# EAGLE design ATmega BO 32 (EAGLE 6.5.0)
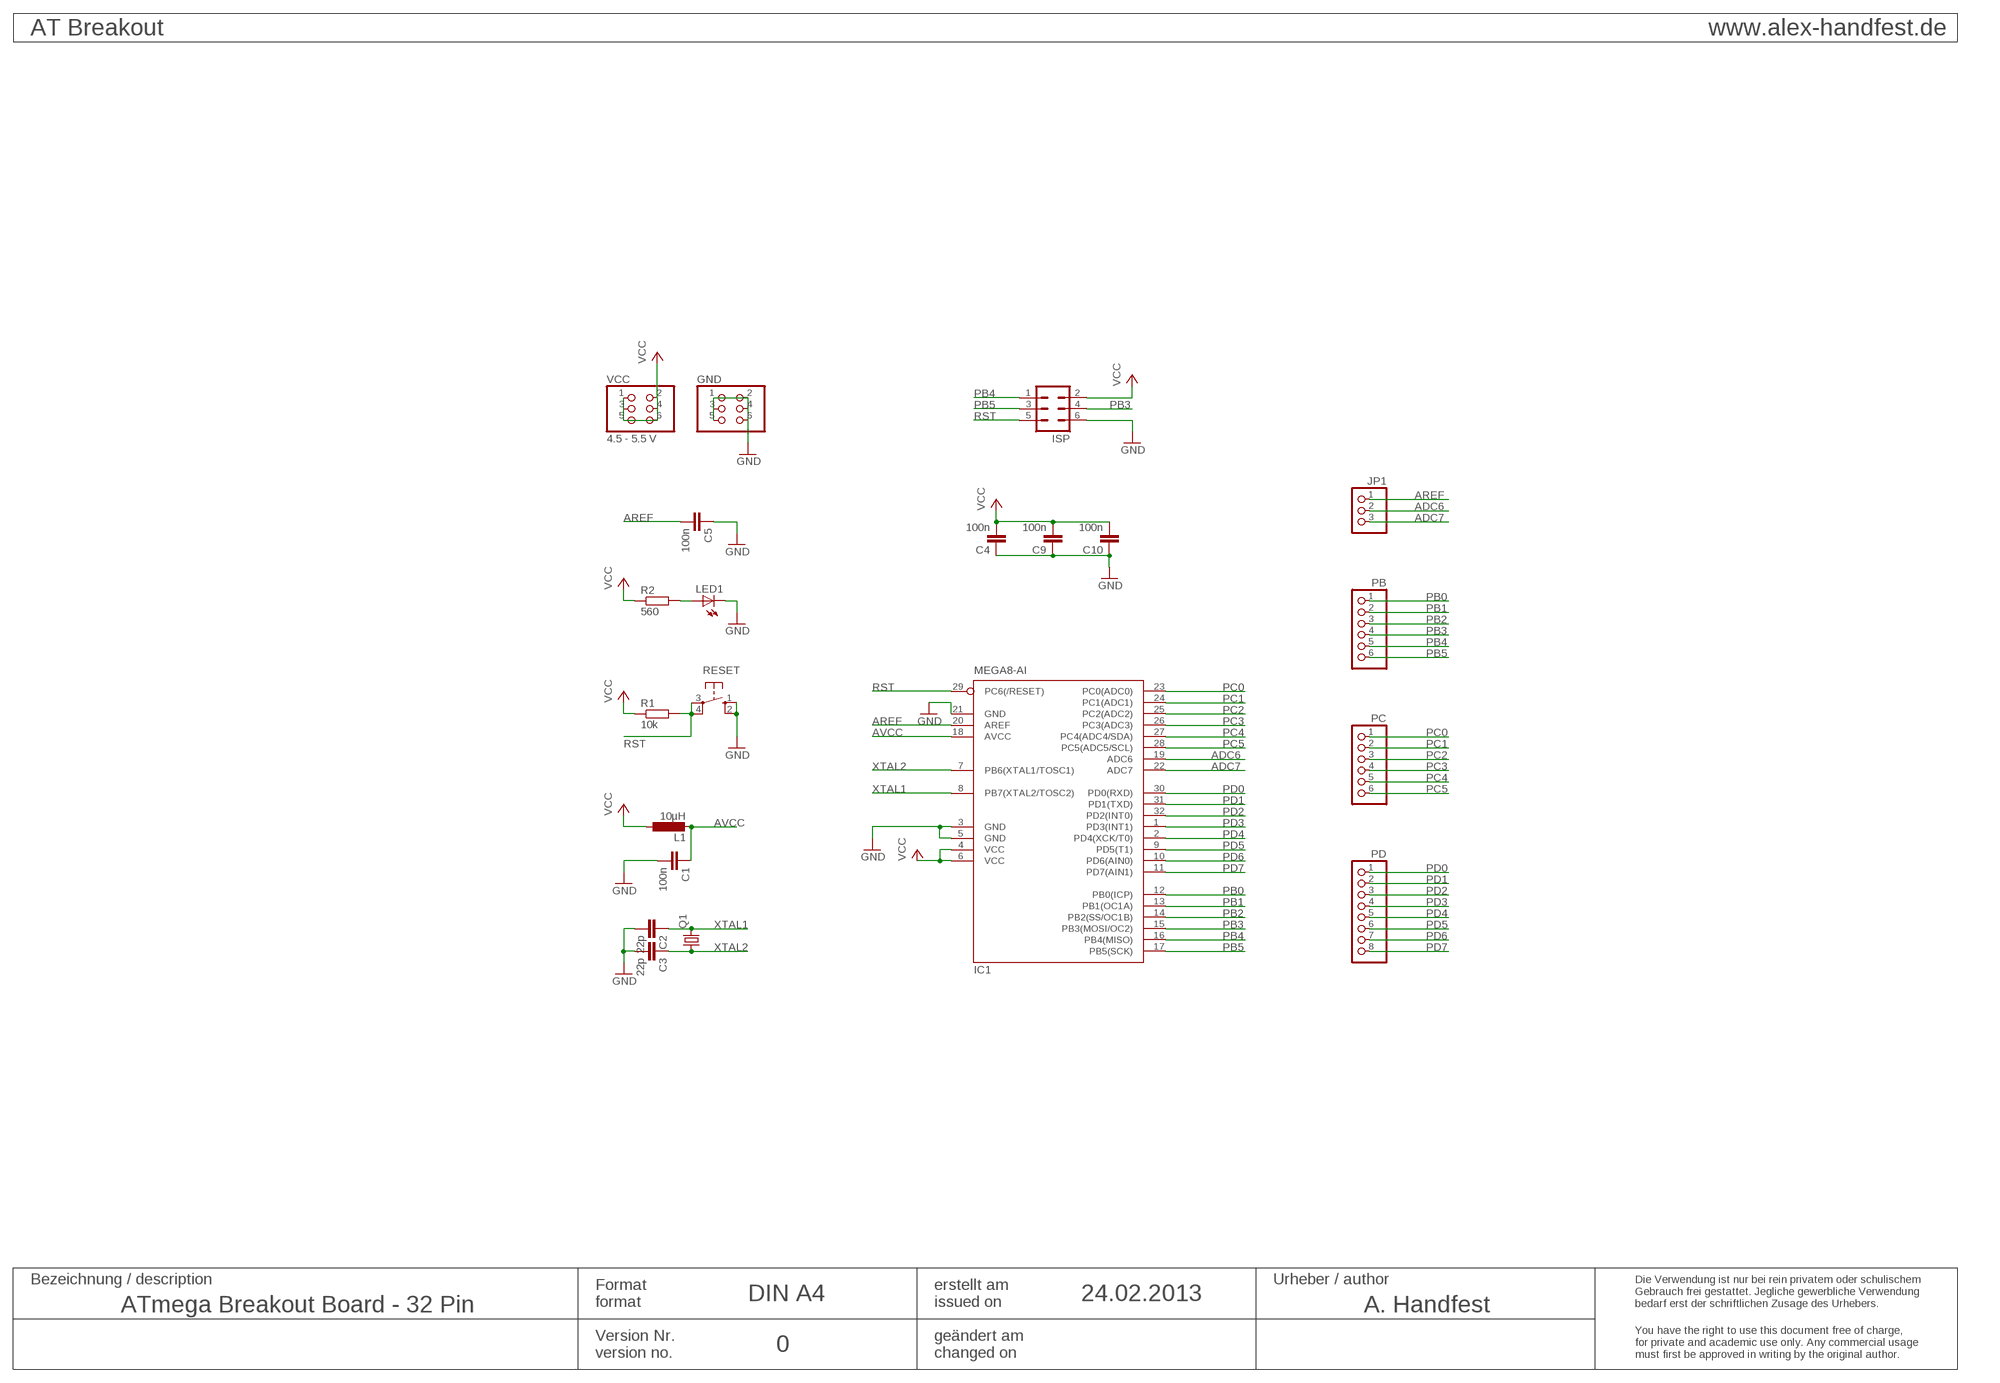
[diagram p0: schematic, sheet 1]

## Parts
C1  100n  C-EUC0805  [C0805]
C2  22p  C-EUC0805  [C0805]
C3  22p  C-EUC0805  [C0805]
C4  100n  C-EUC0805  [C0805]
C5  100n  C-EUC0805  [C0805]
C9  100n  C-EUC0805  [C0805]
C10  100n  C-EUC0805  [C0805]
GND  PINHD-2X3  [2X03]
IC1  MEGA8-AI  [TQFP32-08]
ISP  ML6  [ML6]
JP1  PINHD-1X3  [1X03]
L1  10µH  L-EUL2012C  [L2012C]
LED1  LEDCHIP-LED0805  [CHIP-LED0805]
PB  PINHD-1X6  [1X06]
PC  PINHD-1X6  [1X06]
PD  PINHD-1X8  [1X08]
Q1  CRYSTALCTS406  [CTS406]
R1  10k  R-EU_R0805  [R0805]
R2  560  R-EU_R0805  [R0805]
RESET  10-XX  [B3F-10XX]
VCC  4.5 - 5.5 V  PINHD-2X3  [2X03]

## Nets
ADC6: IC1.19(ADC6) JP1.2
ADC7: IC1.22(ADC7) JP1.3
AREF: C5.2 IC1.20(AREF) JP1.1
AVCC: C1.1 IC1.18(AVCC) L1.2
GND: C1.2 C2.2 C3.2 C4.1 C5.1 C9.1 C10.1 GND.1 GND.2 GND.3 GND.4 GND.5 GND.6 IC1.3(GND) IC1.5(GND) IC1.21(GND) ISP.6 LED1.C RESET.1(S) RESET.2(S1)
N$6: LED1.A R2.2
PB0: IC1.12(PB0(ICP)) PB.1
PB1: IC1.13(PB1(OC1A)) PB.2
PB2: IC1.14(PB2(SS/OC1B)) PB.3
PB3: IC1.15(PB3(MOSI/OC2)) ISP.4 PB.4
PB4: IC1.16(PB4(MISO)) ISP.1 PB.5
PB5: IC1.17(PB5(SCK)) ISP.3 PB.6
PC0: IC1.23(PC0(ADC0)) PC.1
PC1: IC1.24(PC1(ADC1)) PC.2
PC2: IC1.25(PC2(ADC2)) PC.3
PC3: IC1.26(PC3(ADC3)) PC.4
PC4: IC1.27(PC4(ADC4/SDA)) PC.5
PC5: IC1.28(PC5(ADC5/SCL)) PC.6
PD0: IC1.30(PD0(RXD)) PD.1
PD1: IC1.31(PD1(TXD)) PD.2
PD2: IC1.32(PD2(INT0)) PD.3
PD3: IC1.1(PD3(INT1)) PD.4
PD4: IC1.2(PD4(XCK/T0)) PD.5
PD5: IC1.9(PD5(T1)) PD.6
PD6: IC1.10(PD6(AIN0)) PD.7
PD7: IC1.11(PD7(AIN1)) PD.8
RST: IC1.29(PC6(/RESET)) ISP.5 R1.2 RESET.3(P) RESET.4(P1)
VCC: C4.2 C9.2 C10.2 IC1.4(VCC) IC1.6(VCC) ISP.2 L1.1 R1.1 R2.1 VCC.1 VCC.2 VCC.3 VCC.4 VCC.5 VCC.6
XTAL1: C2.1 IC1.8(PB7(XTAL2/TOSC2)) Q1.3
XTAL2: C3.1 IC1.7(PB6(XTAL1/TOSC1)) Q1.1

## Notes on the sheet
- AT Breakout | www.alex-handfest.de
- Bezeichnung / description | Urheber / author
- Format | erstellt am
- DIN A4 | 24.02.2013
- format | issued on
- Die Verwendung ist nur bei rein privatem oder schulischem
  Gebrauch frei gestattet. Jegliche gewerbliche Verwendung 
  bedarf erst der schriftlichen Zusage des Urhebers.
- ATmega Breakout Board - 32 Pin | A. Handfest
- Version Nr. | geändert am
- 0
- version no. | changed on
- You have the right to use this document free of charge,
  for private and academic use only. Any commercial usage
  must first be approved in writing by the original author.

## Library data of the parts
C1-C5 C9 C10 = rcl:C-EU: CAPACITOR, European symbol
GND VCC = pinhead:PINHD-2X3: PIN HEADER
IC1 = atmel:MEGA8: MICROCONTROLLER 8 Kbytes FLASH, 1 kbytes SRAM, 512 bytes EEPROM, USART, 6-channel 10 bit ADC, 2-channel 8 bit ADC Pin compatible with Atmega48, ATMega88, ATMega168 Source: avr.lbr
ISP = con-harting-ml:ML6: HARTING
JP1 = pinhead:PINHD-1X3: PIN HEADER
L1 = rcl:L-EU: INDUCTOR, European symbol
LED1 = led:LED: LED
PB PC = pinhead:PINHD-1X6: PIN HEADER
PD = pinhead:PINHD-1X8: PIN HEADER
Q1 = crystal:CRYSTAL: CRYSTAL; OC_FARNELL: unknown; OC_NEWARK: unknown
R1 R2 = rcl:R-EU_: RESISTOR, European symbol
RESET = switch-omron:10-XX: OMRON SWITCH

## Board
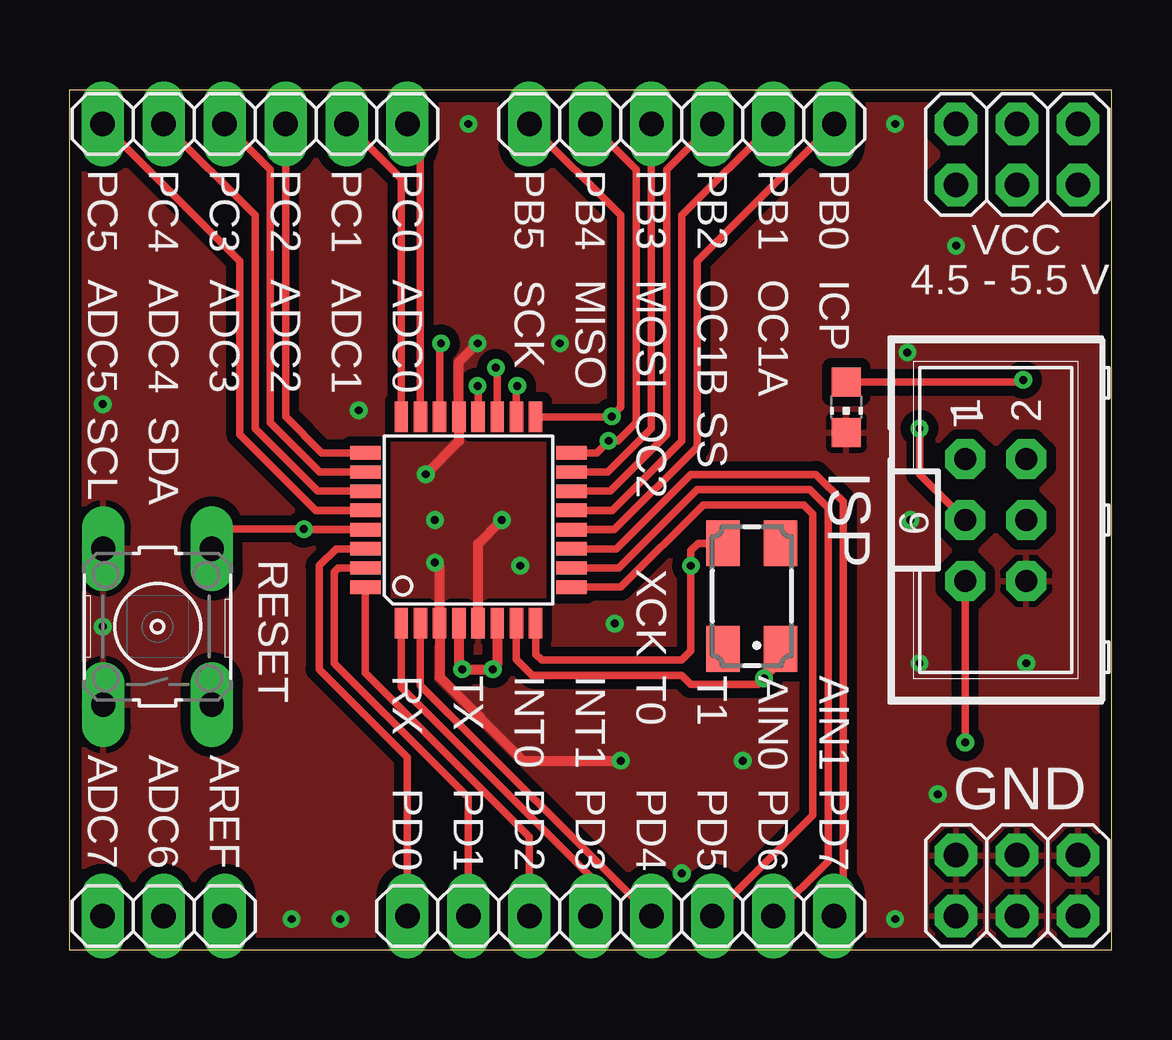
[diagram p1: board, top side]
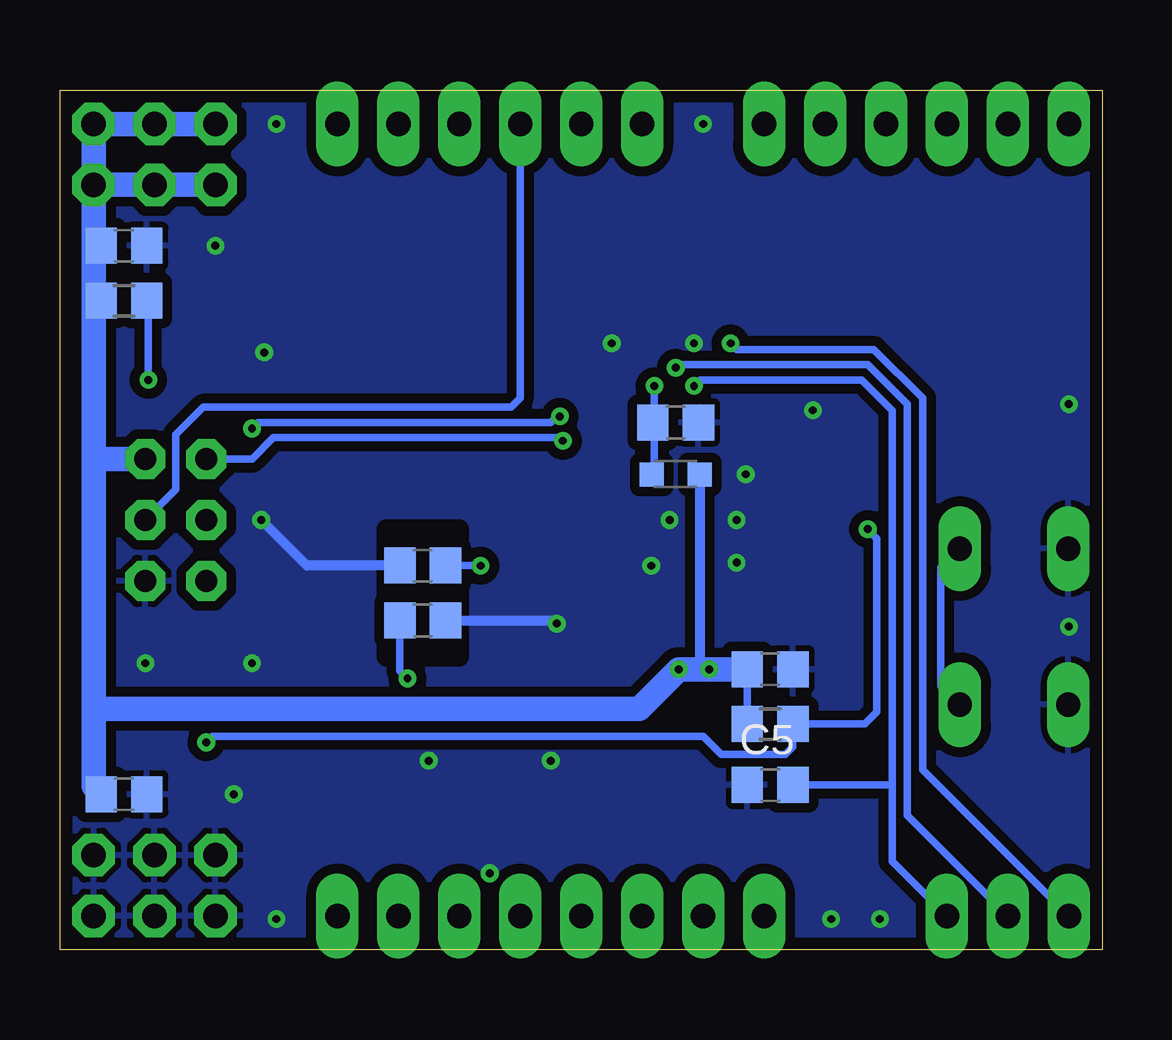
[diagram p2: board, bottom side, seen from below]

Size 43.43 x 35.81 mm. Coordinates in mm from the lower left corner, seen from the top.
Outline: 0,0 43.43,0 43.43,35.81 0,35.81 0,0
Copper layers (1*16): Top 0.035mm / dielectric 1.5mm / Bottom 0.035mm
Design rules "default *": minimum track width 10mil, minimum drill 24mil, track to track 8mil, track to pad 8mil, pad to pad 8mil, via to via 8mil, smd to smd 8mil, copper to edge 20mil, drill to drill 8mil, minimum pad ring 15mil, minimum via ring 8mil, stop-mask expansion 4mil, vias tented up to drill 20mil, thermal gap 10mil
bRestrict: area 26.8,12.2 to 29.8,17.5

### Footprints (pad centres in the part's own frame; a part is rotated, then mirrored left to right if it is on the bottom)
C0805 = smd 1.3 x 1.5: 1 -0.95,0; 2 0.95,0
2X03 = drill 1.016 octagon: 1 -2.54,-1.27; 2 -2.54,1.27; 3 0,-1.27; 4 0,1.27; 5 2.54,-1.27; 6 2.54,1.27
TQFP32-08 = smd 1.27 x 0.559: 1 -4.293,2.8; 2 -4.293,2; 3 -4.293,1.2; 4 -4.293,0.4; 5 -4.293,-0.4; 6 -4.293,-1.2; 7 -4.293,-2; 8 -4.293,-2.8; 17 4.293,-2.8; 18 4.293,-2; 19 4.293,-1.2; 20 4.293,-0.4; 21 4.293,0.4; 22 4.293,1.2; 23 4.293,2; 24 4.293,2.8 | smd 0.559 x 1.27: 9 -2.8,-4.293; 10 -2,-4.293; 11 -1.2,-4.293; 12 -0.4,-4.293; 13 0.4,-4.293; 14 1.2,-4.293; 15 2,-4.293; 16 2.8,-4.293; 25 2.8,4.293; 26 2,4.293; 27 1.2,4.293; 28 0.4,4.293; 29 -0.4,4.293; 30 -1.2,4.293; 31 -2,4.293; 32 -2.8,4.293
ML6 = drill 0.914 octagon: 1 -2.54,-1.27; 2 -2.54,1.27; 3 0,-1.27; 4 0,1.27; 5 2.54,-1.27; 6 2.54,1.27
1X03 = drill 1.016 long: 1 -2.54,0; 2 0,0; 3 2.54,0
L2012C = smd 1 x 1: 1 -1,0; 2 1,0
CHIP-LED0805 = smd 1.2 x 1.2: A 0,-1.05; C 0,1.05
1X06 = drill 1.016 long: 1 -6.35,0; 2 -3.81,0; 3 -1.27,0; 4 1.27,0; 5 3.81,0; 6 6.35,0
1X08 = drill 1.016 long: 1 -8.89,0; 2 -6.35,0; 3 -3.81,0; 4 -1.27,0; 5 1.27,0; 6 3.81,0; 7 6.35,0; 8 8.89,0
CTS406 = smd 1.9 x 1.4: 1 -2.2,-1.2; 2 2.2,-1.2; 3 2.2,1.2; 4 -2.2,1.2
R0805 = smd 1.3 x 1.5: 1 -0.95,0; 2 0.95,0
B3F-10XX = drill 1.016 long: 1 -3.251,2.261; 2 3.251,2.261; 3 -3.251,-2.261; 4 3.251,-2.261

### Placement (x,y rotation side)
C1  17.78,21.97 0 bottom
C2  28.32,16 180 bottom
C3  28.32,13.72 0 bottom
C4  13.84,11.68 180 bottom
C5  13.84,6.86 0 bottom
C9  40.77,6.48 180 bottom
C10  40.77,29.34 180 bottom
GND  39.5,2.67 0 top
IC1  16.64,17.91 90 top
ISP  38.61,17.91 270 top
JP1  3.94,1.4 180 top
L1  17.78,19.81 180 bottom
LED1  32.38,22.61 180 top
PB  25.53,34.42 180 top
PC  7.75,34.42 180 top
PD  22.99,1.4 0 top
Q1  28.45,14.73 90 top
R1  13.84,9.4 0 bottom
R2  40.77,27.05 0 bottom
RESET  3.68,13.46 90 top
VCC  39.5,33.15 0 top

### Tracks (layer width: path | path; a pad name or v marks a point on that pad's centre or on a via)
ADC6  (via drill 0.33)
  Top 0.305: IC1.19 17.84,24.2 v17.78,24.26
  Bottom 0.305: JP1.2 8.13,5.59 8.13,22.73 9.78,24.38 17.65,24.38 v17.78,24.26
ADC7  (via drill 0.33)
  Top 0.305: IC1.22 15.44,25.22 v15.49,25.27
  Bottom 0.305: JP1.3 7.49,7.49 7.49,22.99 9.53,25.02 15.24,25.02 v15.49,25.27
AREF  (via drill 0.33)
  Top 0.305: IC1.20 17.04,23.48 v17.02,23.5
  Bottom 0.305: JP1.1 8.76,3.68 8.76,6.86 | 8.76,6.86 8.76,22.48 10.03,23.75 16.76,23.75 v17.02,23.5 | C5.2 8.76,6.86
AVCC  (via drill 0.33)
  Top 0.305: IC1.18 18.64,23.46 v18.67,23.5
  Bottom 0.305: v18.67,23.5 18.67,21.59 | 18.67,21.59 18.67,19.92 L1.2 | C1.1 18.73,21.65 18.67,21.59
GND  (via drill 0.33)
  Top 0.406: v22.99,7.87 18.92,7.87 15.44,11.36 IC1.3 15.44,15.93 v15.24,16.13 | v17.02,25.27 16.24,24.49 IC1.21 16.24,21.19 v14.86,19.81 | IC1.5 17.04,16.91 v18.03,17.91
  Bottom 0.406: C3.2 22.86,13.72 v22.73,13.59 | C2.2 33.15,16 v35.05,17.91
  other vias: 16.64,34.42 34.42,34.42 34.42,1.27 11.3,1.27 9.27,1.27 36.96,29.34 15.24,17.91 18.8,16 36.2,6.48 39.88,11.94 35.43,11.94 34.92,24.89 25.53,3.17 28.07,7.87 12.06,22.48 20.45,25.27 1.4,22.73 1.4,13.46
  pour Bottom (isolate 0.406): -0.25,-0.25 43.69,-0.25 43.69,36.07 -0.25,36.07
  pour Top (isolate 0.406): -0.25,36.07 43.69,36.07 43.69,-0.25 -0.25,-0.25
N$6  (via drill 0.33)
  Top 0.305: LED1.A 39.66,23.66 v39.75,23.75
  Bottom 0.305: v39.75,23.75 39.75,26.98 R2.2
PB0
  Top 0.305: IC1.12 22.71,17.51 26.16,20.95 26.16,28.7 PB.1
PB1
  Top 0.305: IC1.13 22.62,18.31 25.53,21.21 25.53,30.61 PB.2
PB2
  Top 0.305: IC1.14 22.54,19.11 24.89,21.46 24.89,32.51 PB.3
PB3
  Top 0.305: IC1.15 22.45,19.91 24.26,21.72 PB.4
  Bottom 0.305: PB.4 24.26,22.99 24.64,22.61 37.47,22.61 38.61,21.46 38.61,19.18 ISP.4
PB4  (via drill 0.33)
  Top 0.305: PB.5 23.62,32.51 23.62,21.97 22.86,21.21 v22.48,21.21 21.98,20.71 IC1.16
  Bottom 0.305: ISP.1 35.43,20.45 34.54,21.34 22.61,21.34 v22.48,21.21
PB5  (via drill 0.33)
  Top 0.305: PB.6 22.99,30.61 22.99,22.61 v22.61,22.23 22.58,22.2 IC1.17 | v35.43,21.72 35.43,19.81 ISP.3
  Bottom 0.305: v22.61,22.23 22.73,22.23 22.99,21.97 35.18,21.97 v35.43,21.72
PC0
  Top 0.305: IC1.23 14.64,33.88 PC.1
PC1
  Top 0.305: IC1.24 13.84,32.14 PC.2
PC2
  Top 0.305: IC1.25 10.54,20.71 9.02,22.23 PC.3
PC3
  Top 0.305: IC1.26 10.45,19.91 8.38,21.97 8.38,32.51 PC.4
PC4
  Top 0.305: IC1.27 10.36,19.11 7.75,21.72 7.75,30.61 PC.5
PC5
  Top 0.305: IC1.28 10.27,18.31 7.11,21.46 7.11,28.7 PC.6
PD0
  Top 0.305: IC1.30 11.12,16.71 10.41,16 10.41,11.68 14.1,8 PD.1
PD1
  Top 0.305: IC1.31 11.21,15.91 11.05,15.75 11.05,11.94 16.64,6.35 PD.2
PD2
  Top 0.305: IC1.32 12.34,11.53 19.18,4.7 PD.3
PD3
  Top 0.305: IC1.1 13.84,10.93 21.72,3.05 PD.4
PD4
  Top 0.305: IC1.2 14.64,11.02 PD.5
PD5
  Top 0.305: IC1.9 22.98,15.11 26.42,18.54 30.61,18.54 30.99,18.16 30.99,5.59 PD.6
PD6
  Top 0.305: IC1.10 22.89,15.91 26.16,19.18 30.86,19.18 31.62,18.41 31.62,3.68 PD.7
PD7
  Top 0.305: IC1.11 22.8,16.71 25.91,19.81 31.11,19.81 32.26,18.67 32.26,1.78 PD.8
RST  (via drill 0.33)
  Top 0.305: RESET.4 6.76,17.53 v9.78,17.53 9.8,17.51 IC1.29 | v37.34,8.64 ISP.5
  Bottom 0.305: RESET.3 6.73,11 6.73,15.93 RESET.4 | v9.78,17.53 9.4,17.14 9.4,9.91 9.91,9.4 R1.2 12.89,8.44 13.21,8.13 15.88,8.13 16.64,8.89 37.08,8.89 v37.34,8.64
VCC  (via drill 0.33)
  Top 0.406: IC1.4 16.24,11.83 v16.38,11.68 v17.65,11.68 17.84,11.87 IC1.6
  Bottom 0.305: C10.2 42.04,29.34 | R1.1 C4.2 | R2.1 41.91,27.05 42.04,26.92
  Bottom 0.406: L1.1 16.78,11.79 16.89,11.68
  Bottom 1.016: VCC.5 42.04,29.34 42.04,26.92 42.04,20.45 | 42.04,20.45 42.04,10.03 | 42.04,10.03 42.04,6.8 C9.2 | ISP.2 42.04,20.45 | VCC.1 VCC.3 VCC.5 | VCC.2 VCC.4 VCC.6 VCC.5 | 42.04,10.03 19.3,10.03 v17.65,11.68 16.89,11.68 v16.38,11.68 C4.2
XTAL1  (via drill 0.33)
  Top 0.305: IC1.8 19.44,12.31 19.68,12.06 25.53,12.06 25.91,12.45 v25.91,16 25.91,16.64 26.2,16.93 Q1.3
  Bottom 0.305: v25.91,16 C2.1
XTAL2  (via drill 0.33)
  Top 0.305: IC1.7 18.64,12.1 19.3,11.43 25.53,11.43 25.91,11.05 28.7,11.05 v28.96,11.3 29.65,11.99 Q1.1
  Bottom 0.305: C3.1 29.27,11.62 v28.96,11.3

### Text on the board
tNames: PC5 | PC4 | PC3 | PC2 | PC1 | PC0 | PB5 | PB4 | PB3 | PB2 | PB1 | PB0 | ADC5 | ADC4 | ADC3 | ADC2 | ADC1 | ADC0 | SCK | MISO | MOSI | OC1B | OC1A | ICP | 1 | SCL | SDA | OC2 | SS | XCK | RX | TX | INT0 | INT1 | T0 | T1 | AIN0 | AIN1 | ADC7 | ADC6 | AREF | PD0 | PD1 | PD2 | PD3 | PD4 | PD5 | PD6 | PD7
